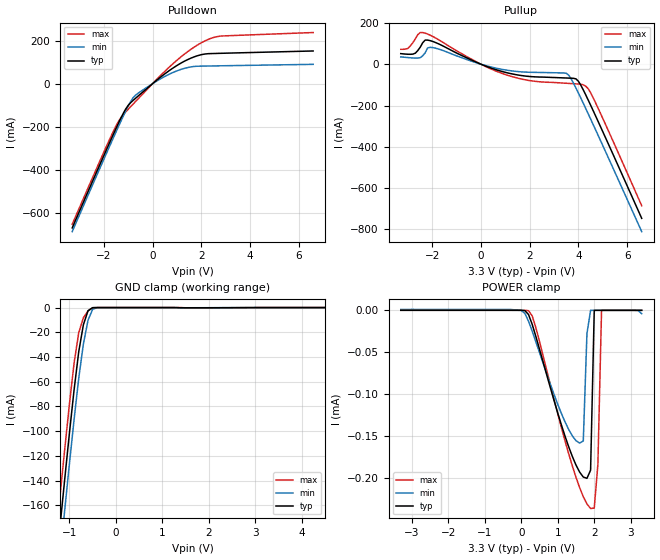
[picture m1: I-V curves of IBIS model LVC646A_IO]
|TEXAS INSTRUMENTS INCORPORATED
|Standard Linear and Logic Group
|IBIS Model of LVC646A
|Octal Registered Transceiver with 3-State Outputs
|SSOP 24-pin (DB), SOP 24-pin (DW), TSSOP 24-pin (PW) Package
[IBIS Ver]   2.1
[Comment char]  |_char
[File Name]   lvc646a.ibs
[File Rev]   1.0
[Date]   10/20/97
[Source]   File originated at Texas Instruments, Inc.
[Notes]   The following is an IBIS list for the LVC646A.
|   - All test data contained in this file are derived from
|   hspice(tm) simulations.
|   - File created by Ramzi Ammar, SLL Applications
|   - This file may be incomplete or may not be fully compliant
|   with the IBIS specification. It will be replaced with a
|   version that is IBIS Revision 3.2 compliant and is complete
|   and accurate.
|   Please email all questions and comments to sllibis@ti.com.
[Disclaimer] Property of Texas Instruments Incorporated.  Unauthorized
   reproduction and/or distribution is strictly prohibited.
   This product is protected under copyright law.
   Created 1997, (C) Copyright 1997, Texas Instruments Inc.,
   All Rights Reserved
   UNLESS THERE IS A SIGNED, WRITTEN AGREEMENT TO THE
   CONTRARY, TEXAS INSTRUMENTS ("TI") IS PROVIDING THE IBIS
   MODELS "AS IS" AND WITHOUT ANY WARRANTY, EXPRESSED OR
   IMPLIED.  TI assumes no liability for:
   1) the accuracy of the IBIS models provided to your
   company;
   2) the proper functioning of these IBIS models in your
   design or for any resulting applications; or
   3) infringement of patents, copyrights or intellectual
   property rights resulting from your use of these IBIS
   models.
   TI provides IBIS Models as a service to our customers.
   You and your company shall not distribute, sell or give
   these models to anyone else without prior written
   permission from TI.
   TI reserves the right to make changes to our products or
   to discontinue any semiconductor product or service
   without notice, and advises our customers to obtain the
   latest version of relevant information to verify, before
   placing orders, that the information being relied on is
   current.
   Please be aware that your receipt and use of the IBIS
   information provided shall serve as acceptance of these
   terms and conditions.  If you do not accept these terms,
   you should return or destroy the IBIS models and any
   other accompanying information immediately.
[Component]   LVC646A_DB
[Manufacturer]  Texas Instruments, Inc.
[Package]
|	  typ 	min   max
R_pkg	  0.045	0.04   0.049
L_pkg	  3.668nH	3.226nH	4.415nH
C_pkg	  0.416pF	0.349pF	0.507pF
[Pin]	signal_name	model_name	 R_pin	L_pin   C_pin
1   CLKAB	NC   0.042	4.299nH	0.503pF
2   SAB	NC   0.04   3.96nH	0.499pF
3   DIR	NC   0.042	3.775nH	0.417pF
4   A1	LVC646A_IO	 0.047	3.487nH	0.369pF
5   A2   LVC646A_IO	 0.046	3.347nH	0.352pF
6   A3	LVC646A_IO	 0.049	3.352nH	0.371pF
7   A4	LVC646A_IO	 0.046	3.226nH	0.363pF
8   A5	LVC646A_IO	 0.047	3.289nH	0.349pF
9   A6	LVC646A_IO	 0.047	3.347nH	0.361pF
10   A7	LVC646A_IO	 0.041	3.576nH	0.409pF
11   A8	LVC646A_IO   0.041	3.995nH	0.503pF
12   GND	GND   0.045	4.415nH	0.507pF
13   B8	LVC646A_IO   0.043	4.337nH	0.506pF
14   B7	LVC646A_IO   0.042	4.003nH	0.504pF
15   B6	LVC646A_IO   0.041	3.686nH	0.41pF
16   B5	LVC646A_IO	 0.048	3.355nH	0.349pF
17   B4	LVC646A_IO	 0.047	3.301nH	0.353pF
18   B3	LVC646A_IO	 0.048	3.268nH	0.366pF
19   B2	LVC646A_IO	 0.048	3.269nH	0.366pF
20   B1	LVC646A_IO	 0.047	3.314nH	0.349pF
21   OE	NC   0.048	3.399nH	0.355pF
22   SBA	NC   0.041	3.688nH	0.412pF
23   CLKBA	NC   0.042	4.003nH	0.504pF
24   VCC	POWER   0.043	4.347nH	0.505pF
|   Component LVC646A_DW
[Component]   LVC646A_DW
[Manufacturer]  Texas Instruments, Inc.
[Package]
|   typ   min   max
R_pkg   0.037	0.03   0.047
L_pkg   5.146nH  3.993nH	6.885nH
C_pkg   0.758pF  0.512pF	1.067pF
[Pin]	signal_name	model_name	 R_pin	L_pin   C_pin
1   CLKAB	NC   0.039	6.885nH	1.067pF
2   SAB	NC   0.042	5.95nH	0.958pF
3   DIR	NC   0.047	5.317nH	0.791pF
4   A1	LVC646A_IO	 0.031	4.651nH	0.611pF
5   A2	LVC646A_IO	 0.03   3.993nH	0.512pF
6   A3	LVC646A_IO	 0.03   4.083nH	0.611pF
7   A4	LVC646A_IO	 0.03   4.083nH	0.611pF
8   A5	LVC646A_IO	 0.03   3.993nH	0.512pF
9   A6	LVC646A_IO   0.031	4.652nH	0.611pF
10   A7	LVC646A_IO   0.047	5.317nH	0.791pF
11   A8	LVC646A_IO   0.042	5.95nH	0.959pF
12   GND	GND   0.039	6.885nH	1.067pF
13   B8	LVC646A_IO   0.039	6.885nH	1.067pF
14   B7	LVC646A_IO   0.042	5.95nH	0.959pF
15   B6	LVC646A_IO   0.047	5.317nH	0.791pF
16   B5	LVC646A_IO	 0.031	4.652nH	0.611pF
17   B4	LVC646A_IO	 0.03   3.993nH	0.512pF
18   B3	LVC646A_IO	 0.03   4.083nH	0.61pF
19   B2	LVC646A_IO	 0.03   4.083nH	0.61pF
20   B1	LVC646A_IO	 0.03   3.993nH	0.512pF
21   OE	NC   0.031	4.651nH	0.611pF
22   SBA	NC   0.047	5.317nH	0.791pF
23   CLKBA	NC   0.042	5.95nH	0.958pF
24   VCC	POWER   0.039	6.885nH	1.067pF
|   Component LVC646A_PW
[Component]   LVC646A_PW
[Manufacturer]  Texas Instruments, Inc.
[Package]
|		typ   min	max
R_pkg		0.039   0.03	0.046
L_pkg		2.685nH  2.367nH	3.177nH
C_pkg		0.32pF   0.252pF	0.434pF
[Pin]	signal_name	model_name	 R_pin 	L_pin   C_pin
1   CLKAB	NC   0.037	3.153nH	0.434pF
2   SAB	NC   0.034	2.629nH	0.341pF
3   DIR	NC   0.032	2.86nH	0.347pF
4   A1	LVC646A_IO	 0.042	2.741nH	0.29pF
5   A2   LVC646A_IO	 0.046	2.6nH   0.262pF
6   A3	LVC646A_IO	 0.043	2.414nH	0.266pF
7   A4	LVC646A_IO	 0.042	2.367nH	0.262pF
8   A5   LVC646A_IO	 0.044	2.461nH	0.252pF
9   A6	LVC646A_IO   0.042	2.543nH	0.274pF
10   A7	LVC646A_IO   0.03   2.616nH	0.332pF
11   A8	LVC646A_IO   0.037	2.67nH	0.346pF
12   GND	GND   0.039	3.177nH	0.433pF
13   B8	LVC646A_IO   0.037	3.111nH	0.431pF
14   B7 	LVC646A_IO   0.037	2.656nH	0.345pF
15   B6	LVC646A_IO   0.031	2.739nH	0.34pF
16   B5	LVC646A_IO	 0.042	2.649nH	0.282pF
17   B4	LVC646A_IO	 0.046	2.532nH	0.257pF
18   B3	LVC646A_IO	 0.044	2.425nH	0.266pF
19   B2	LVC646A_IO	 0.044	2.425nH	0.266pF
20   B1	LVC646A_IO	 0.046	2.532nH	0.257pF
21   OE   NC   0.042	2.648nH	0.282pF
22   SBA	NC   0.031	2.738nH	0.339pF
23   CLKBA	NC   0.036	2.653nH	0.344pF
24   VCC	POWER   0.037	3.11nH	0.431pF
| Models and submodels in the file (1): LVC646A_IO (I/O)
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|   Model LVC646A_IO
[Model]   LVC646A_IO
Model_type   I/O
Polarity   Inverting
Enable   Active-Low
Vinl = 0.8V
Vinh = 2.0V
|variable   typ   min   max
C_comp   7.5pF   NA   NA
[Voltage range]   3.3   3.0   3.6
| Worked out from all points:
|   slope of the pulldown table from 0 to 0.495 V, typ, clamps not added: 11 ohm
|   slope of the pullup table from 0 to 0.495 V, typ, clamps not added: 22.7 ohm
|   GND clamp passes 1 mA (typ) near -0.54 V on its own axis
[Pullup]   | Note: Vtable = Vcc - Voutput
|   Voltage   I(typ)   I(min)   I(max)
-3.3V     51.6mA     35.88mA    72.42mA
-3V       48.59mA    32.37mA    77.34mA
-2.7V     53.82mA    29.98mA    123.8mA
-2.4V     104.1mA    40.75mA    153.8mA
-2.2V     117.2mA    78.97mA    146.6mA
-2V       111.2mA    81.18mA    135.7mA
900mV     -36.21mA   -25.52mA   -45.85mA
2V        -59.23mA   -38.84mA   -79.22mA
3.5V      -66.61mA   -43.71mA   -92.1mA
4V        -82.56mA   -139.7mA   -95.77mA
4.4V      -173.1mA   -239.8mA   -118.5mA
6.6V      -747.2mA   -811.6mA   -686mA
[Pulldown]
|   Voltage   I(typ)   I(min)   I(max)
-3.3V     -667.5mA   -684.7mA   -650.8mA
-1.5V     -207.3mA   -223.3mA   -195.4mA
-1.3V     -159.4mA   -173.9mA   -157.3mA
-1.1V     -116.6mA   -126.1mA   -130.4mA
-800mV    -77.43mA   -65.31mA   -94.48mA
-600mV    -57.81mA   -44.52mA   -70.78mA
400mV     36.73mA    27.26mA    45.85mA
1.1V      91mA       63.71mA    117.9mA
1.8V      127.9mA    80.82mA    176mA
2.4V      139.6mA    82.23mA    210.1mA
2.9V      141.1mA    83.21mA    221.3mA
6.6V      151.7mA    89.79mA    237mA
[GND_Clamp]
|   Voltage   I(typ)   I(min)   I(max)
-3.3V     -1.009A    -1.033A    -985.8mA
-1.3V     -214.2mA   -239.3mA   -189.7mA
-1.2V     -175.9mA   -201mA     -151.5mA
-1.1V     -138.2mA   -163.3mA   -114mA
-1V       -101.5mA   -126.2mA   -77.91mA
-900mV    -66.49mA   -90.46mA   -44.84mA
-800mV    -35.67mA   -57.14mA   -20.29mA
-700mV    -13.84mA   -29.32mA   -8.191mA
-600mV    -2.515mA   -10.19mA   -2.697mA
-500mV    -71.34uA   -1.341mA   -142.5uA
-300mV    -90.6nA    -4.019uA   -513nA
6.6V      45.46nA    1.093uA    15.11nA
[POWER_Clamp]   | Note: Vtable = Vcc - Voutput
|   Voltage   I(typ)   I(min)   I(max)
-3.3V     45.46nA    1.092uA    15.8nA
-100mV    16.6nA     426.1nA    9.053nA
200mV     -5.058uA   -13.02uA   -398.5nA
1.1V      -136.8uA   -123.2uA   -140.1uA
1.6V      -193.2uA   -158.6uA   -211.8uA
1.7V      -199.1uA   -156uA     -222.6uA
1.8V      -200.7uA   -27.73uA   -231.2uA
1.9V      -190.9uA   -3.627nA   -236.7uA
2V        -4.778nA   -4.02nA    -236.2uA
2.1V      -2.779nA   -4.424nA   -183.9uA
2.2V      -3.066nA   -4.828nA   -21.34nA
3.3V      -6.227nA   -4.019uA   -5.96nA
[Ramp]
|Variable   typ   min   max
dV/dt_r   1.2865E+00/8.3194E-10  9.9193E-01/1.3869E-09  1.5294E+00/5.8528E-10
dV/dt_f   1.6230E+00/3.3814E-09  1.3743E+00/7.7278E-09  1.8424E+00/1.7861E-09
